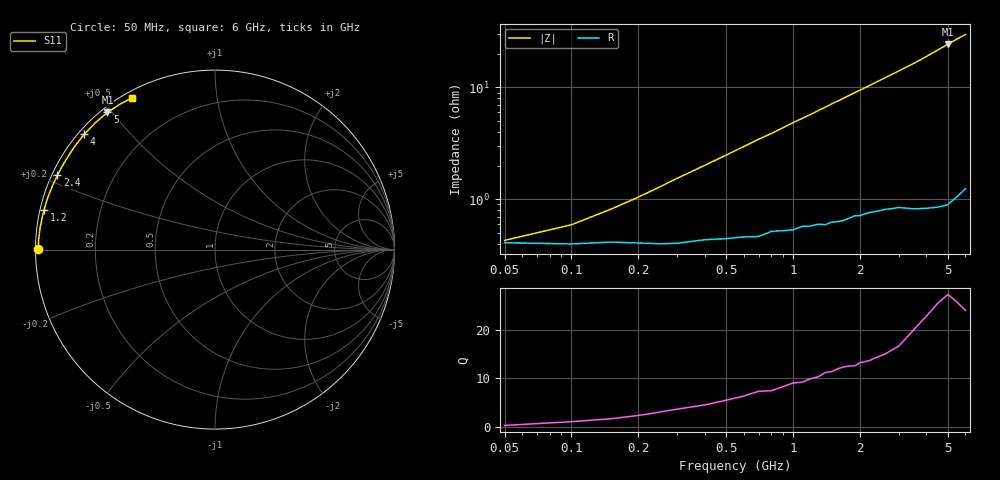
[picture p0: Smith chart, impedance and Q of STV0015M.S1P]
! SIEMENS Discrete & RF Semiconductors
! BA892
! Si PIN Diode in SCD-80
! IF = 15 mA
! S-Parameters:  September  1997
# GHz  S  MA  R  50
!  f  S11
! GHz  MAG  ANG
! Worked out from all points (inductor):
!   34 points, 50 MHz to 6 GHz, reference 50 ohm
!   read as one part to ground: L = 782 pH near 250 MHz
!   highest Q = 25.6 at 5 GHz (marker M1), where L = 774 pH
!   S11 on the Smith chart (normalised r, x): 50 MHz: 0.01, +0.00; 1.2 GHz: 0.01, +0.11; 2.4 GHz: 0.02, +0.22; 4 GHz: 0.02, +0.38; 5 GHz: 0.02, +0.49; 6 GHz: 0.02, +0.59
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0.05  0.9838 179.7
0.1  0.9842 179.0
0.15  0.9836 178.4
0.25  0.9841 177.2
0.3  0.984 176.6
0.5  0.9824 174.4
0.7  0.9817 172.2
0.8  0.9797 171.2
1  0.9791 169.0
1.1  0.9776 168.0
1.2  0.9775 167.0
1.3  0.9767 165.9
1.4  0.977 164.9
1.5  0.9758 163.8
1.6  0.9756 162.8
1.7  0.975 161.8
1.8  0.9739 160.7
1.9  0.9728 159.7
2  0.9728 158.7
2.4  0.9707 154.7
2.8  0.9696 150.7
3  0.9691 148.7
3.5  0.9708 143.8
4  0.9714 138.6
4.5  0.9717 133.3
5  0.9715 128.1
5.5  0.9679 123.1
6  0.964 118.5
